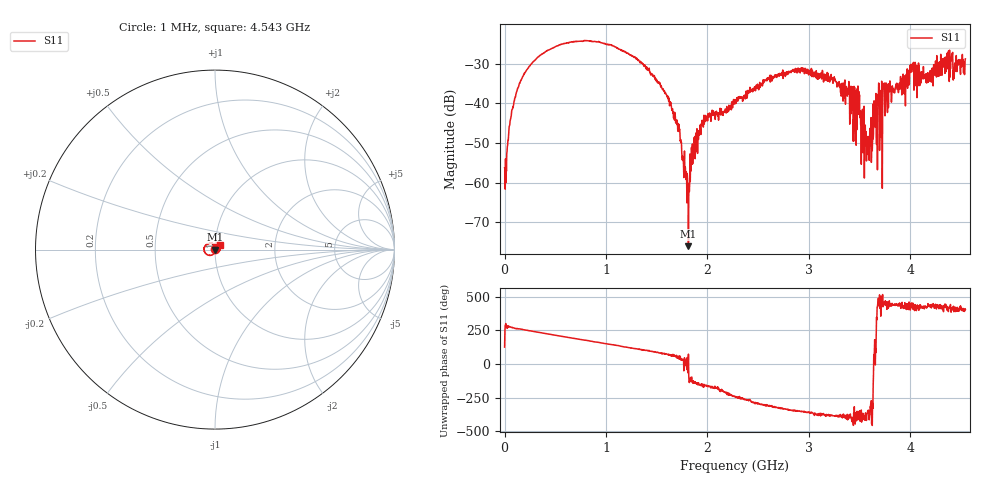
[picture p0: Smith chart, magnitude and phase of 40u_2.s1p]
# HZ S RI R 50
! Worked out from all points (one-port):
!   1515 points, 1 MHz to 4.543 GHz, reference 50 ohm
!   lowest |S11| = -76.0 dB at 1.813 GHz (marker M1), VSWR 1.00, Z = 50 + j0.0152 ohm
!   |S11| at or under -10 dB: start of sweep to end of sweep
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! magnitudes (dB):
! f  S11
! 1 MHz  -56.3
! 67 MHz  -43.0
! 166 MHz  -34.0
! 343 MHz  -28.1
! 571 MHz  -25.1
! 1.138 GHz  -26.4
! 1.531 GHz  -34.8
! 1.705 GHz  -44.9
! 1.798 GHz  -65.1
! 1.813 GHz  -76.0
! 1.855 GHz  -55.2
! 1.96 GHz  -46.0
! 2.272 GHz  -39.7
! 2.842 GHz  -31.9
! 3.241 GHz  -34.3
! 3.409 GHz  -42.8
! 3.451 GHz  -36.0
! 3.49 GHz  -42.8
! 3.529 GHz  -41.5
! 3.589 GHz  -48.4
! 3.643 GHz  -39.4
! 3.718 GHz  -34.4
! 3.748 GHz  -40.8
! 3.976 GHz  -34.3
! 4.012 GHz  -30.2
! 4.162 GHz  -34.9
! 4.36 GHz  -27.4
! 4.543 GHz  -28.8
